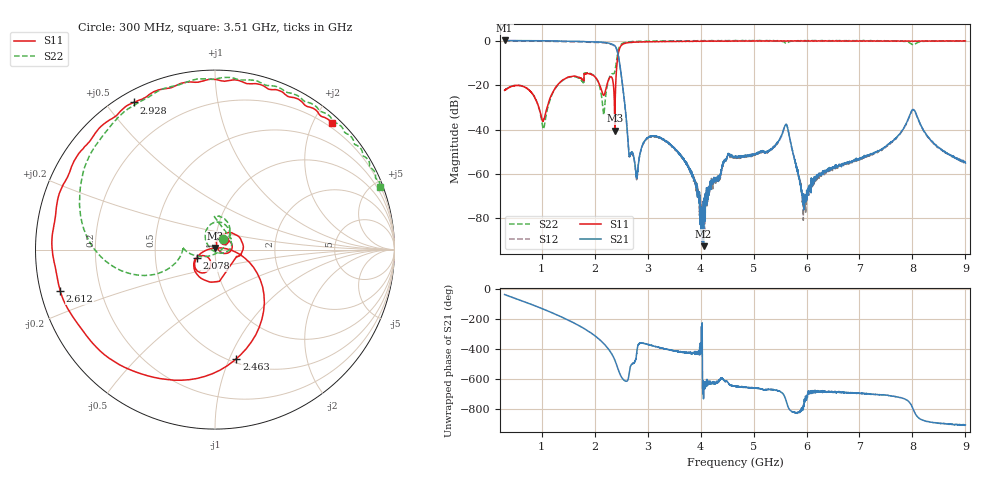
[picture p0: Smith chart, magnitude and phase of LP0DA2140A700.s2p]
!Agilent Technologies,E8358A,US41080443,A.07.50.56
!Agilent E8358A: A.07.50.56
!Date: Friday, August 05, 2016 08:40:27
!Correction: S11(Full 2 Port(1,2))
!S21(Full 2 Port(1,2))
!S12(Full 2 Port(1,2))
!S22(Full 2 Port(1,2))
!S2P File: Measurements: S11, S21, S12, S22:Log Frequency Sweep
# Hz S  dB  R 50
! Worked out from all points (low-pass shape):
!   6401 points, 300 MHz to 9 GHz, reference 50 ohm
!   highest |S21| = 0.06 dB at 300.3 MHz (marker M1); lowest = -92.5 dB at 4.055 GHz (marker M2)
!   |S21| within 3 dB of the highest: start of sweep to 2.4 GHz
!   lowest |S11| = -40.6 dB at 2.381 GHz (marker M3), VSWR 1.02, Z = 50.2 + j0.915 ohm
!   |S11| at or under -10 dB: start of sweep to 2.424 GHz
!   |S22| runs from -39.7 to 0.1 dB; largest |S21 - S12| = 0.028
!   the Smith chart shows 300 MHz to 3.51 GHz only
!   S11 on the Smith chart (normalised r, x): 300 MHz: 1.10, +0.12; 2.078 GHz: 0.81, -0.08; 2.463 GHz: 0.54, -1.06; 2.612 GHz: 0.06, -0.13; 2.928 GHz: 0.04, +0.59; 3.51 GHz: 0.14, +2.30
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3e8  -22.38 47.0  0.05 -38.4  -0.18 -38.3  -22.38 53.0
3.00319e8  -22.37 47.0  0.06 -38.4  -0.17 -38.3  -22.39 52.9
1.032672e9  -35.87 35.1  -0.07 -135.6  -0.30 -135.4  -39.58 -118.0
1.21374e9  -23.11 71.5  -0.12 -162.3  -0.35 -162.1  -23.32 137.5
1.75044e9  -17.13 -14.6  -0.38 106.0  -0.61 106.1  -17.90 49.2
2.078239e9  -18.98 -155.9  -0.64 27.1  -0.88 27.3  -19.40 40.2
2.173115e9  -24.63 -129.2  -0.79 -4.5  -1.02 -4.3  -33.32 -68.8
2.381115e9  -40.57 76.5  -2.31 -113.5  -2.54 -113.4  -13.89 -167.5
2.463495e9  -4.16 -78.9  -9.00 165.5  -9.17 165.6  -3.13 176.7
2.611798e9  -0.99 -165.0  -39.26 107.0  -39.55 107.3  -0.70 116.5
2.785265e9  -0.65 147.3  -60.40 -90.4  -60.92 -90.6  -0.34 84.6
2.927937e9  -0.57 118.9  -45.74 -3.3  -46.11 -3.2  -0.31 66.5
3.201372e9  -0.52 79.0  -43.52 -29.2  -43.60 -27.7  -0.21 41.6
3.509656e9  -0.39 46.9  -48.39 -52.3  -48.70 -52.9  -0.17 20.5
4.05548e9  -0.30 11.3  -92.49 -11.0  -75.31 55.5  -0.05 -4.5
4.651453e9  -0.17 -11.6  -52.14 74.3  -52.91 76.8  0.03 -22.5
5.599354e9  -0.23 -33.7  -38.10 -7.3  -38.27 -6.6  -1.09 -44.3
5.923832e9  -0.20 -39.4  -70.34 -66.1  -70.98 -83.2  -0.09 -44.7
6.102778e9  -0.11 -42.5  -63.47 38.9  -64.17 29.1  0.03 -48.2
7.552286e9  -0.24 -70.6  -46.35 10.8  -46.82 9.6  -0.13 -78.3
8.028242e9  -0.29 -80.2  -31.15 -90.7  -31.36 -90.7  -1.91 -86.1
9e9  -0.19 -98.1  -55.09 175.2  -54.77 175.0  -0.18 -111.8
